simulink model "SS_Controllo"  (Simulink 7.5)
settings: Solver=FixedStepDiscrete  StartTime=0.0  StopTime=10.0  FixedStep=Ts  RelTol=1e-3
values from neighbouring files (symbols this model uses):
  As1 = 1    [TSC160720ProvaMatlab.m]
  As2 = 2    [TSC160720ProvaMatlab.m]
  Kff = -inv(Cz*inv(Az-Bz*K-eye(n))*Bz)    [TSC160720ProvaMatlab.m]
  ts1 = 0    [TSC160720ProvaMatlab.m]
  ts2 = 5    [TSC160720ProvaMatlab.m]
  X0 = [0, 0, 0]'    [TSC160720ProvaMatlab.m]
undefined symbols (not defined in the file or in its folder): Az, Bz, Cz, K
libraries: simulink x1

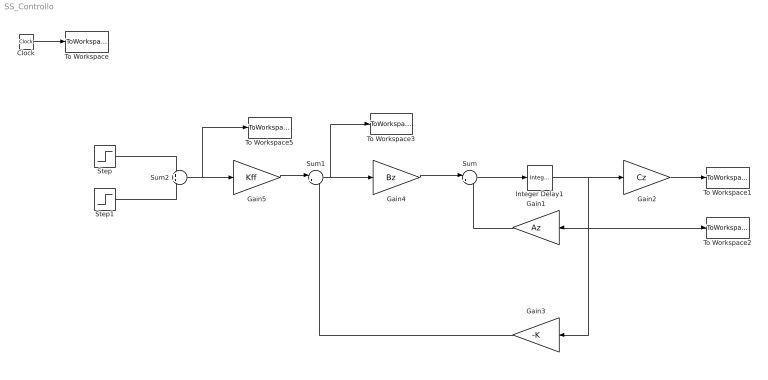
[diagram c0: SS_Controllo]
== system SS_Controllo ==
  Clock : Clock
  Gain1 : Gain  Gain=Az  Multiplication=Matrix(K*u)
  Gain2 : Gain  Gain=Cz  Multiplication=Matrix(K*u)
  Gain3 : Gain  Gain=-K  Multiplication=Matrix(K*u)
  Gain4 : Gain  Gain=Bz  Multiplication=Matrix(K*u)
  Gain5 : Gain  Gain=Kff  Multiplication=Matrix(K*u)
  Integer Delay1 : simulink/Discrete/Integer Delay  vinit=X0  samptime=Ts  NumDelays=1
  Step : Step  Time=ts1  After=As1  SampleTime=0
  Step1 : Step  Time=ts2  After=As2  SampleTime=0
  Sum : Sum  Inputs=|++
  Sum1 : Sum  Inputs=|++
  Sum2 : Sum
  To Workspace : ToWorkspace  VariableName=time  SampleTime=-1  SaveFormat=Array
  To Workspace1 : ToWorkspace  VariableName=y  SampleTime=-1  SaveFormat=Array
  To Workspace2 : ToWorkspace  VariableName=X  SampleTime=-1  SaveFormat=Array
  To Workspace3 : ToWorkspace  VariableName=u  SampleTime=-1  SaveFormat=Array
  To Workspace5 : ToWorkspace  VariableName=yref  SampleTime=-1  SaveFormat=Array
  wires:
  Gain1/1 -> Sum/2
  Sum/1 -> Integer Delay1/1
  Integer Delay1/1 -> Gain2/1, Gain1/1, To Workspace2/1, Gain3/1
  Gain2/1 -> To Workspace1/1
  Gain4/1 -> Sum/1
  Clock/1 -> To Workspace/1
  Gain5/1 -> Sum1/1
  Sum1/1 -> Gain4/1, To Workspace3/1
  Gain3/1 -> Sum1/2
  Step/1 -> Sum2/1
  Sum2/1 -> To Workspace5/1, Gain5/1
  Step1/1 -> Sum2/2
